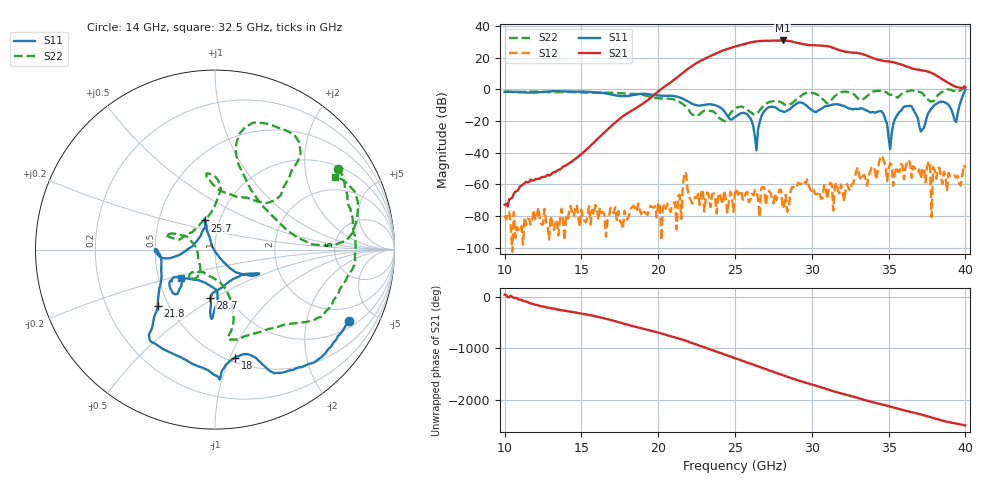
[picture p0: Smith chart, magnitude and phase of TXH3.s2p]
!Keysight Technologies,M9808A,MY58100618,A.14.70.03
!Date: Monday, February 27, 2023 13:18:24
!Correction: S11(C  2-Port  )
!S21(C  2-Port  )
!S12(C  2-Port  )
!S22(C  2-Port  )
!S2P File: Measurements: S11, S21, S12, S22:
# Hz S  RI  R 50
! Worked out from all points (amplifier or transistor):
!   301 points, 10 GHz to 40 GHz, reference 50 ohm
!   highest |S21| = 30.9 dB at 28.1 GHz (marker M1)
!   |S21| within 3 dB of that: 25.32 GHz to 29.87 GHz (4.553 GHz wide, 16.5 % of centre)
!   unconditionally stable (mu >= 1): start of sweep to 39.78 GHz
!   at 15 GHz: K = 37211.71, MAG = -31.2 dB, |S12| = -76.1 dB
!   at 25 GHz: K = 39.49, MAG = 27.3 dB, |S12| = -65.6 dB
!   at 40 GHz: K = -2.86, MSG = 25.6 dB, |S12| = -49.8 dB
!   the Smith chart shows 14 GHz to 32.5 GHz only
!   S11 on the Smith chart (normalised r, x): 14 GHz: 1.27, -3.56; 18 GHz: 0.54, -1.04; 21.8 GHz: 0.43, -0.34; 25.7 GHz: 0.85, +0.28; 28.7 GHz: 0.82, -0.48; 32.5 GHz: 0.66, -0.22
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1e10  0.7562 0.3348  0.000158 0.000161  0.000105 -3.73e-06  0.0244 0.8558
1.4e10  0.7453 -0.3996  0.000269 0.00391  -1.79e-05 -8.79e-05  0.6847 0.4518
1.5e10  0.6117 -0.5816  0.00721 0.00528  -0.000123 9.87e-05  0.7368 0.3051
1.8e10  0.1116 -0.6014  -0.1754 0.00545  -6.6e-05 3.73e-05  0.6871 -0.2447
2e10  -0.1598 -0.6165  0.7723 0.3652  -0.00015 -0.000177  0.2328 -0.4641
2.18e10  -0.3186 -0.3154  -2.772 -2.796  -0.00196 0.00147  0.0833 -0.2705
2.33e10  -0.3353 0.000965  3.986 9.936  0.0003 0.000303  -0.1295 -0.1658
2.41e10  -0.2497 -0.0478  15.34 -4.291  0.000219 0.000253  -0.0928 -0.0631
2.5e10  -0.0603 0.118  -8.359 -20.67  -5.48e-05 -0.000525  -0.2174 0.0866
2.57e10  -0.056 0.1622  -27.57 2.782  -0.000517 -0.000112  -0.2415 0.0653
2.66e10  0.0505 -0.0723  8.182 32.42  -4.53e-05 7.97e-05  -0.0198 0.2098
2.74e10  0.2471 -0.1328  33.88 -5.116  -0.000285 -0.000261  -0.00984 0.4142
2.81e10  0.1311 -0.1512  5.143 -34.51  4.7e-05 -0.000163  -0.0131 0.364
2.87e10  -0.0259 -0.2692  -26.35 -18.93  -0.000339 -0.000726  0.2362 0.2679
2.92e10  -0.0186 -0.3863  -27.65 5.939  -0.00102 -0.000146  0.4102 0.395
3e10  0.00396 -0.2212  -2.886 24.43  6.18e-05 0.000604  0.3042 0.6991
3.1e10  -0.2394 -0.1767  23.05 1.173  -0.000115 0.000314  0.2569 0.2515
3.16e10  -0.2362 -0.2408  10.94 -15.06  -0.000182 0.00111  0.6553 0.0232
3.25e10  -0.1868 -0.1585  -8.373 -11.89  0.000476 -0.000416  0.6668 0.407
3.37e10  -0.1963 -0.0332  -7.348 8.228  7.19e-05 0.00182  0.627 -0.2602
3.5e10  -0.0273 -0.0136  6.227 4.263  -0.0018 -0.00245  0.6958 0.1313
4e10  0.4485 -0.8759  1.105 0.3711  0.00324 5.51e-05  1.193 -0.6024
